(* Logix 5000 AddOnInstructionDefinition export AMCI_SMD23E2_Run_Blend_Move; software revision 20.03 *)

ADD_ON_INSTRUCTION AMCI_SMD23E2_Run_Blend_Move   (* revision 1.0, vendor AMCI *)
VAR_INPUT
   Type_0_for_standard_1_for_indexed : BOOL;
   Direction_0_for_CW_1_for_CCW : BOOL; {required}
END_VAR
VAR_IN_OUT
   AMCI_SMD23E2_output_data : _000A:SMD23E2_788832CB:O:0; {required}
END_VAR
VAR
   command_data_block : INT[10];
        [0]   // Command Bits MSW
        [1]   // Command Bits LSW
        [2]   // Upper Target Position
        [3]   // Lower Target Position
        [4]   // Upper Programmed Speed
        [5]   // Lower Programmed Speed
END_VAR

ROUTINE Logic   (* ladder *)
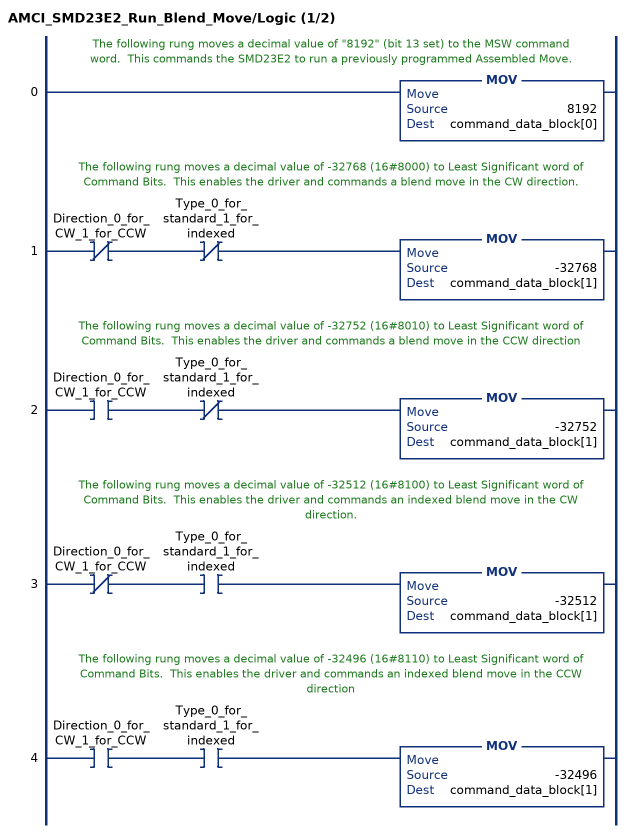
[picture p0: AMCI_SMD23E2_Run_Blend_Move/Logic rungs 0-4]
   // The following rung moves a decimal value of "8192" (bit 13 set) to the MSW command word.  This commands the SMD23E2 to run a previously programmed Assembled Move.
   0: MOV(8192,command_data_block[0]);
   // The following rung moves a decimal value of -32768 (16#8000) to Least Significant word of Command Bits.  This enables the driver and commands a blend move in the CW direction.
   1: XIO(Direction_0_for_CW_1_for_CCW)XIO(Type_0_for_standard_1_for_indexed)MOV(-32768,command_data_block[1]);
   // The following rung moves a decimal value of -32752 (16#8010) to Least Significant word of Command Bits.  This enables the driver and commands a blend move in the CCW direction
   2: XIC(Direction_0_for_CW_1_for_CCW)XIO(Type_0_for_standard_1_for_indexed)MOV(-32752,command_data_block[1]);
   // The following rung moves a decimal value of -32512 (16#8100) to Least Significant word of Command Bits.  This enables the driver and commands an indexed blend move in the CW direction.
   3: XIO(Direction_0_for_CW_1_for_CCW)XIC(Type_0_for_standard_1_for_indexed)MOV(-32512,command_data_block[1]);
   // The following rung moves a decimal value of -32496 (16#8110) to Least Significant word of Command Bits.  This enables the driver and commands an indexed blend move in the CCW direction
   4: XIC(Direction_0_for_CW_1_for_CCW)XIC(Type_0_for_standard_1_for_indexed)MOV(-32496,command_data_block[1]);
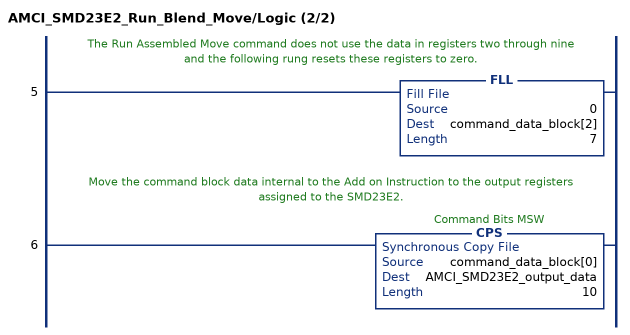
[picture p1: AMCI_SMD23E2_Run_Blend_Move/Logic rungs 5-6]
   // The Run Assembled Move command does not use the data in registers two through nine and the following rung resets these registers to zero.
   5: FLL(0,command_data_block[2],7);
   // Move the command block data internal to the Add on Instruction to the output registers assigned to the SMD23E2.
   6: CPS(command_data_block[0],AMCI_SMD23E2_output_data,10);
END_ROUTINE
END_ADD_ON_INSTRUCTION
